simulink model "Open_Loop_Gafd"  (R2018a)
settings: Solver=ode45  StartTime=0.0  StopTime=80  RelTol=1e-3  EnableMultiTasking=on
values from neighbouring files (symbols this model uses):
  Cyb = -0.0245    [init.m]    (also in lqr_des.m)
  Cydel = [-0.24668,0.24668, 0.47413,-0.47413,0]/100    [init.m]    (also in lqr_des.m = [-0.24668,0.24668, 0.47413,-0.47413]/100)
  Cza = -0.073    [init.m]
  Czdel = [0.51664,0.51664,0.60478,0.60478,0.06]/100    [init.m]
  d2r = pi/180    (= 0.0174532925199)    [init.m]
  Mass = 198.32    [init.m]    (also in lqr_des.m)
  Qbar = 150    [init.m]    (also in lqr_des.m)
  r2d = 180/pi    (= 57.2957795131)    [init.m]    (also in pl.m)
  Sref = 79.069    [init.m]    (also in lqr_des.m)
  V0 = 822.8    [init.m]
undefined symbols (not defined in the file or in its folder): Abfp, Afla, Ardr, Avf, Bbfp, Bfla, Brdr, Bvf, Cbfp, Cfla, Crdr, Cvf, Dbfp, Dfla, Drdr, Dvf, K4axmix, Kpr, Kq

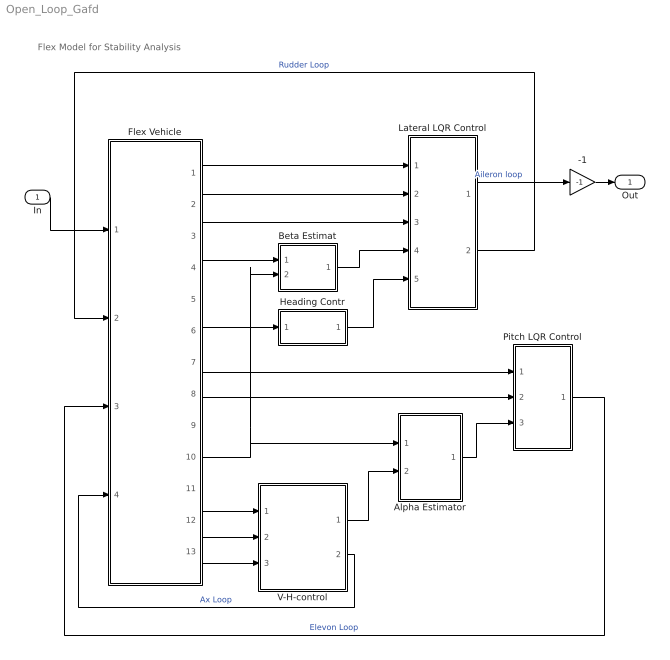
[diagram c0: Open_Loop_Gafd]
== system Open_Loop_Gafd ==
  note: Flex Model for Stability Analysis
  In : Inport
  -1 : Gain  Gain=-1
  Alpha Estimator : Subsystem
  Beta Estimat : Subsystem
  Flex Vehicle : Subsystem
  Heading Contr : Subsystem
  Lateral LQR Control : Subsystem
  Pitch LQR Control : Subsystem
  V-H-control : Subsystem
  Out : Outport
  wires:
  Flex Vehicle/2(p) -> Lateral LQR Control/2(p)
  Flex Vehicle/3(r) -> Lateral LQR Control/3(r)
  Flex Vehicle/1(phi) -> Lateral LQR Control/1(phi)
  Flex Vehicle/8(q) -> Pitch LQR Control/2(q)
  Flex Vehicle/7(thet) -> Pitch LQR Control/1(thet)
  Flex Vehicle/4(Ny) -> Beta Estimat/1(Ydd)
  Flex Vehicle/6("chi ") -> Heading Contr/1(chi)
  Flex Vehicle/12(Nz) -> V-H-control/2(Az)
  Flex Vehicle/13(dH) -> V-H-control/3(dH)
  Flex Vehicle/11(V-dot) -> V-H-control/1(Vdot)
  Flex Vehicle/10(delt) -> Beta Estimat/2(delta), Alpha Estimator/1(delta)
  Alpha Estimator/1(alphat) -> Pitch LQR Control/3(alfa)
  V-H-control/1(Zdd-com) -> Alpha Estimator/2(Zdd)
  Beta Estimat/1(bethat) -> Lateral LQR Control/4(bet)
  -1/1 -> Out/1
  V-H-control/2(Throtle) -> Flex Vehicle/4(Ax-cmd)  "Ax Loop"
  Pitch LQR Control/1(dQ) -> Flex Vehicle/3(dQ)  "Elevon Loop"
  Lateral LQR Control/2(dR) -> Flex Vehicle/2(dR)  "Rudder Loop"
  Heading Contr/1(phi-cmd) -> Lateral LQR Control/5(ph-cmd)
  In/1 -> Flex Vehicle/1(dP)
  Lateral LQR Control/1(dP) -> -1/1  "Aileron loop"

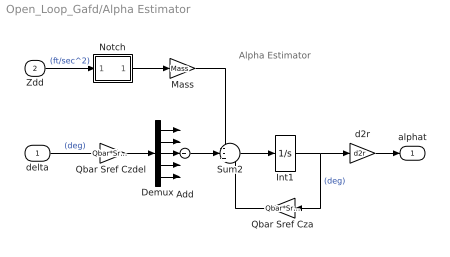
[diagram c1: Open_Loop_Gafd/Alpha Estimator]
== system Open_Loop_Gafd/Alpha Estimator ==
  note: Alpha Estimator
  delta : Inport
  Zdd : Inport  Port=2
  Add : Sum  Inputs=+++++
  Demux : Demux  Outputs=5
  Int1 : Integrator
  Mass : Gain  Gain=Mass
  Notch : Subsystem
  Qbar Sref Cza : Gain  Gain=Qbar*Sref*Cza
  "Qbar Sref Czdel " : Gain  Gain=Qbar*Sref*Czdel
  Sum2 : Sum  Inputs=--+
  d2r : Gain  Gain=d2r
  alphat : Outport
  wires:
  Demux/5 -> Add/5
  Demux/4 -> Add/4
  Demux/3 -> Add/3
  Demux/2 -> Add/2
  Demux/1 -> Add/1
  "Qbar Sref Czdel "/1 -> Demux/1
  delta/1 -> "Qbar Sref Czdel "/1  "(deg)"
  Sum2/1 -> Int1/1
  Int1/1 -> d2r/1, Qbar Sref Cza/1  "(deg)"
  Qbar Sref Cza/1 -> Sum2/3
  Mass/1 -> Sum2/1
  d2r/1 -> alphat/1
  Add/1 -> Sum2/2
  Zdd/1 -> Notch/1(in)  "(ft/sec^2)"
  Notch/1(ou) -> Mass/1

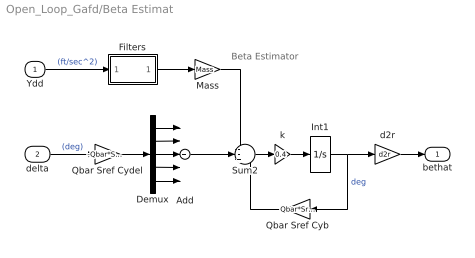
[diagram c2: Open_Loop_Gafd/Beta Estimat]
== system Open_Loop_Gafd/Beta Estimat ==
  note: Beta Estimator
  Ydd : Inport
  delta : Inport  Port=2
  Add : Sum  Inputs=+++++
  Demux : Demux  Outputs=5
  Filters : Subsystem
  Int1 : Integrator
  Mass : Gain  Gain=Mass
  Qbar Sref Cyb : Gain  Gain=Qbar*Sref*Cyb
  Qbar Sref Cydel : Gain  Gain=-Qbar*Sref*Cydel
  Sum2 : Sum  Inputs=--+
  d2r : Gain  Gain=d2r
  k : Gain  Gain=0.4
  bethat : Outport
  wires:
  Filters/1(Ou) -> Mass/1
  Demux/5 -> Add/5
  Demux/4 -> Add/4
  Demux/3 -> Add/3
  Demux/2 -> Add/2
  Demux/1 -> Add/1
  Qbar Sref Cydel/1 -> Demux/1
  delta/1 -> Qbar Sref Cydel/1  "(deg)"
  Sum2/1 -> k/1
  Qbar Sref Cyb/1 -> Sum2/3
  Ydd/1 -> Filters/1(In)  "(ft/sec^2)"
  Mass/1 -> Sum2/1
  d2r/1 -> bethat/1
  Add/1 -> Sum2/2
  Int1/1 -> Qbar Sref Cyb/1, d2r/1  "deg"
  k/1 -> Int1/1

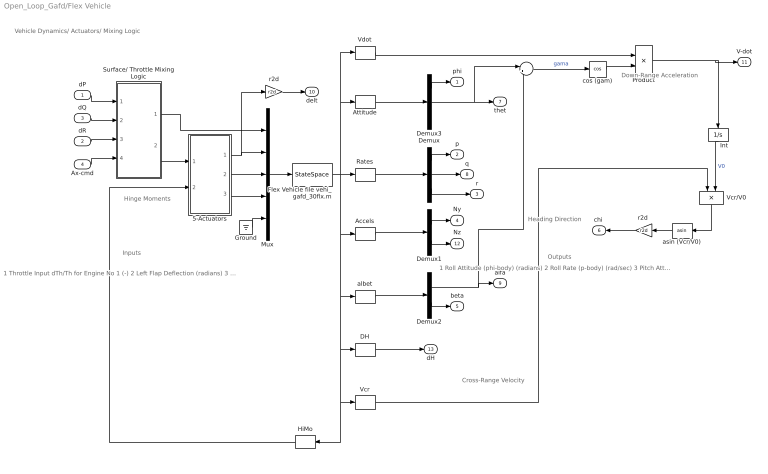
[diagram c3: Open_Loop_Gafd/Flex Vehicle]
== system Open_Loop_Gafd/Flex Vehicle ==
  note: Vehicle Dynamics/ Actuators/ Mixing Logic
  note: Cross-Range Velocity
  note: Heading Direction
  note: Down-Range Acceleration
  note: Outputs
  note: Inputs
  note: 1 Throttle Input dTh/Th for Engine No 1 (-) 2 Left Flap Deflection (radians) 3 Right Flap Deflection (radians) 4 Left Rudder Deflection (radians) 5 Right Rudder Deflection (radians) 6 Body Flap Deflection (radians) 7 Left Flap Velocity (rad/sec) 8 Right Flap Velocity (rad/sec) 9 Left Rudder Velocity (rad/sec) 10 Right Rudder Velocity (rad/sec) 11 Body Flap Velocity (rad/sec) 12 Left Flap Acceleration (rad/s^2) 13 Right Flap Acceleration (rad/s^2) 14 Left Rudder Acceleration (rad/s^2) 15 Right Rudder Acceleration (rad/s^2) 16 Body Flap Acceleration (rad/s^2) 17 Wind Gust Azim, Elev Angles=(45.0 90.0) (deg)
  note: 1 Roll Attitude (phi-body) (radians) 2 Roll Rate (p-body) (rad/sec) 3 Pitch Attitude (thet-bdy) (radians) 4 Pitch Rate (q-body) (rad/sec) 5 Yaw Attitude (psi-body) (radians) 6 Yaw Rate (r-body) (rad/sec) 7 Angle of attack, alfa, (radians) 8 Angle of sideslip, beta, (radian) 9 Change in Altitude, delta-h, (feet) 10 Forward Acceleration (V-dot) (ft/sec) 11 Cross Range Velocity (Vcr) (ft/sec) 12 Rate-Gyro # 1, Roll Rate (Body) (rad/sec) 13 Rate-Gyro # 2, Pitch Rate (Body) (rad/sec) 14 Rate-Gyro # 3, Yaw Rate (Body) (rad/sec) 15 Accelerom # 1, (along Y), (ft/sec^2) Translat. Acceler 16 Accelerom # 2, (along Z), (ft/sec^2) Translat. Acceler 17 Hinge Moment for Aero Surface # 1, (ft-lb) 18 Hinge Moment for Aero Surface # 2, (ft-lb) 19 Hinge Moment for Aero Surface # 3, (ft-lb) 20 Hinge Moment for Aero Surface # 4, (ft-lb) 21 Hinge Moment for Aero Surface # 5, (ft-lb)
  note: Hinge Moments
  dP : Inport
  dR : Inport  Port=2
  dQ : Inport  Port=3
  Ax-cmd : Inport  Port=4
  "    " : Sum  Inputs=|+-
  5-Actuators : Subsystem
  Accels : Selector  InputPortWidth=21  IndexOptions=Index vector (dialog)  Indices=[15,16]  OutputSizes=1
  Attitude : Selector  InputPortWidth=21  IndexOptions=Index vector (dialog)  Indices=[1,3,5]  OutputSizes=1
  DH : Selector  InputPortWidth=21  IndexOptions=Index vector (dialog)  Indices=[9]  OutputSizes=1
  Demux : Demux  Outputs=3
  Demux1 : Demux  Outputs=2
  Demux2 : Demux  Outputs=2
  Demux3 : Demux  Outputs=3
  Flex Vehicle file vehi_gafd_30flx.m : StateSpace  A=Avf  B=Bvf  C=Cvf  D=Dvf  InitialCondition=0
  Ground : Ground
  HiMo : Selector  InputPortWidth=21  IndexOptions=Index vector (dialog)  Indices=[17:21]  OutputSizes=1
  Int : Integrator  InitialCondition=V0
  Mux : Mux  Inputs=[1, 5,5,5, 1]
  Product : Product
  Rates : Selector  InputPortWidth=21  IndexOptions=Index vector (dialog)  Indices=[12:14]  OutputSizes=1
  Surface/ Throttle Mixing Logic : Subsystem
  Vcr : Selector  InputPortWidth=21  IndexOptions=Index vector (dialog)  Indices=[11]  OutputSizes=1
  Vcr/V0 : Product  Inputs=*/
  Vdot : Selector  InputPortWidth=21  IndexOptions=Index vector (dialog)  Indices=[10]  OutputSizes=1
  albet : Selector  InputPortWidth=21  IndexOptions=Index vector (dialog)  Indices=[7,8]  OutputSizes=1
  asin (Vcr/V0) : Trigonometry  Operator=asin
  cos (gam) : Trigonometry  Operator=cos
  r2d : Gain  Gain=r2d
  "r2d " : Gain  Gain=r2d
  phi : Outport
  p : Outport  Port=2
  r : Outport  Port=3
  Ny : Outport  Port=4
  beta : Outport  Port=5
  "chi " : Outport  Port=6
  thet : Outport  Port=7
  q : Outport  Port=8
  alfa : Outport  Port=9
  delt : Outport  Port=10
  V-dot : Outport  Port=11
  Nz : Outport  Port=12
  dH : Outport  Port=13
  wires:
  Vcr/1 -> Vcr/V0/1
  Vdot/1 -> Product/1
  cos (gam)/1 -> Product/2
  DH/1 -> dH/1
  Demux3/1 -> phi/1
  Demux3/2 -> thet/1, "    "/1
  Attitude/1 -> Demux3/1
  Demux2/2 -> beta/1
  Demux2/1 -> alfa/1, "    "/2
  albet/1 -> Demux2/1
  Demux1/2 -> Nz/1
  Demux1/1 -> Ny/1
  Accels/1 -> Demux1/1
  Demux/3 -> r/1
  Demux/2 -> q/1
  Demux/1 -> p/1
  HiMo/1 -> 5-Actuators/2(HM)
  Flex Vehicle file vehi_gafd_30flx.m/1 -> Rates/1, Attitude/1, Vdot/1, Accels/1, albet/1, DH/1, HiMo/1, Vcr/1
  Rates/1 -> Demux/1
  5-Actuators/2(del-dot) -> Mux/3
  5-Actuators/3(del-ddot) -> Mux/4
  5-Actuators/1(delta) -> r2d/1, Mux/2
  Surface/ Throttle Mixing Logic/2(delta) -> 5-Actuators/1(del-cmd)
  "    "/1 -> cos (gam)/1  "gama"
  Int/1 -> Vcr/V0/2  "V0"
  Product/1 -> Int/1, V-dot/1
  asin (Vcr/V0)/1 -> "r2d "/1
  Vcr/V0/1 -> asin (Vcr/V0)/1
  "r2d "/1 -> "chi "/1
  r2d/1 -> delt/1
  Ax-cmd/1 -> Surface/ Throttle Mixing Logic/4(Ax)
  dR/1 -> Surface/ Throttle Mixing Logic/3(yaw)
  dQ/1 -> Surface/ Throttle Mixing Logic/2(ptch)
  dP/1 -> Surface/ Throttle Mixing Logic/1(roll)
  Surface/ Throttle Mixing Logic/1(Throt) -> Mux/1
  Mux/1 -> Flex Vehicle file vehi_gafd_30flx.m/1
  Ground/1 -> Mux/5

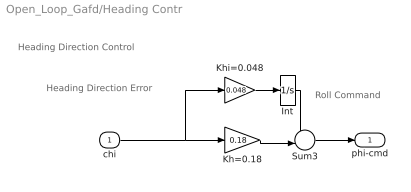
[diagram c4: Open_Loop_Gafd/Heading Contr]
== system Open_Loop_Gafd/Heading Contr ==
  note: Roll Command
  note: Heading Direction Control
  note: Heading Direction Error
  chi : Inport
  Int : Integrator
  Kh=0.18 : Gain  Gain=0.18
  Khi=0.048 : Gain  Gain=0.048
  Sum3 : Sum  Inputs=--|
  phi-cmd : Outport
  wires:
  Khi=0.048/1 -> Int/1
  Kh=0.18/1 -> Sum3/2
  Int/1 -> Sum3/1
  Sum3/1 -> phi-cmd/1
  chi/1 -> Kh=0.18/1, Khi=0.048/1

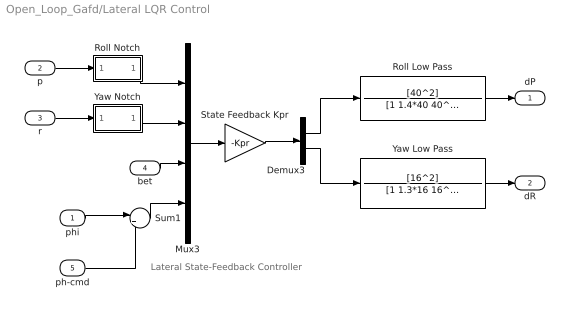
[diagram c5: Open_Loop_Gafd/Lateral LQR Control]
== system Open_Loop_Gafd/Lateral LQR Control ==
  note: Lateral State-Feedback Controller
  phi : Inport
  p : Inport  Port=2
  r : Inport  Port=3
  bet : Inport  Port=4
  ph-cmd : Inport  Port=5
  Demux3 : Demux  Outputs=2
  Mux3 : Mux
  Roll Low Pass : TransferFcn  Numerator=[40^2]  Denominator=[1 1.4*40 40^2]
  Roll Notch : Subsystem
  State Feedback Kpr : Gain  Gain=-Kpr  Multiplication=Matrix(K*u) (u vector)
  Sum1 : Sum  Inputs=|+-
  Yaw Low Pass : TransferFcn  Numerator=[16^2]  Denominator=[1 1.3*16 16^2]
  Yaw Notch : Subsystem
  dP : Outport
  dR : Outport  Port=2
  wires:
  Roll Low Pass/1 -> dP/1
  Demux3/2 -> Yaw Low Pass/1
  r/1 -> Yaw Notch/1(In)
  Roll Notch/1(ou) -> Mux3/1
  ph-cmd/1 -> Sum1/2
  phi/1 -> Sum1/1
  Sum1/1 -> Mux3/4
  Demux3/1 -> Roll Low Pass/1
  bet/1 -> Mux3/3
  p/1 -> Roll Notch/1(in)
  Mux3/1 -> State Feedback Kpr/1
  State Feedback Kpr/1 -> Demux3/1
  Yaw Low Pass/1 -> dR/1
  Yaw Notch/1(Ot) -> Mux3/2

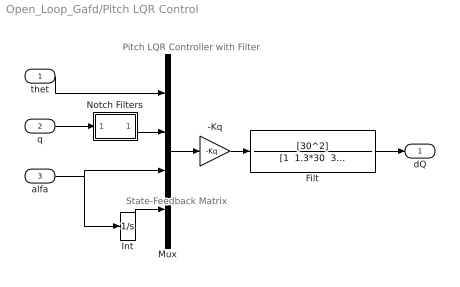
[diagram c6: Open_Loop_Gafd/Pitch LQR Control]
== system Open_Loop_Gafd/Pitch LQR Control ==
  note: State-Feedback Matrix
  note: Pitch LQR Controller with Filter
  thet : Inport
  q : Inport  Port=2
  alfa : Inport  Port=3
  -Kq : Gain  Gain=-Kq  Multiplication=Matrix(K*u)
  Filt : TransferFcn  Numerator=[30^2]  Denominator="[1  1.3*30  30^2]"
  Int : Integrator
  Mux : Mux
  Notch Filters : Subsystem
  dQ : Outport
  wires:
  Filt/1 -> dQ/1
  Notch Filters/1(ou) -> Mux/2
  alfa/1 -> Int/1, Mux/3
  thet/1 -> Mux/1
  q/1 -> Notch Filters/1(in)
  -Kq/1 -> Filt/1
  Int/1 -> Mux/4
  Mux/1 -> -Kq/1

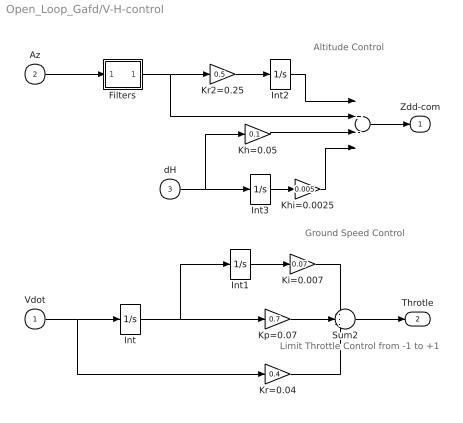
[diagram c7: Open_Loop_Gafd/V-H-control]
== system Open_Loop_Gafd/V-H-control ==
  note: Limit Throttle Control from -1 to +1
  note: Ground Speed Control
  note: Altitude Control
  Vdot : Inport
  Az : Inport  Port=2
  dH : Inport  Port=3
  "  " : Sum  Inputs=++--
  Filters : Subsystem
  Int{,1..3} (4 alike) : Integrator
  Kh=0.05 : Gain  Gain=0.1
  Khi=0.0025 : Gain  Gain=0.005
  Ki=0.007 : Gain  Gain=0.07
  Kp=0.07 : Gain  Gain=0.7
  Kr2=0.25 : Gain  Gain=0.5
  Kr=0.04 : Gain  Gain=0.4
  Sum2 : Sum  Inputs=---
  Zdd-com : Outport
  Throtle : Outport  Port=2
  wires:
  Khi=0.0025/1 -> "  "/4
  Int3/1 -> Khi=0.0025/1
  "  "/1 -> Zdd-com/1
  Int2/1 -> "  "/1
  Kr2=0.25/1 -> Int2/1
  Kh=0.05/1 -> "  "/3
  dH/1 -> Kh=0.05/1, Int3/1
  Int/1 -> Int1/1, Kp=0.07/1
  Int1/1 -> Ki=0.007/1
  Ki=0.007/1 -> Sum2/1
  Kp=0.07/1 -> Sum2/2
  Kr=0.04/1 -> Sum2/3
  Sum2/1 -> Throtle/1
  Vdot/1 -> Kr=0.04/1, Int/1
  Filters/1(ou) -> "  "/2, Kr2=0.25/1
  Az/1 -> Filters/1(in)

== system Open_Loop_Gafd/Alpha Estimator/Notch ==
  note: Notch Filters
  in : Inport
  Notch 79 rad : TransferFcn  Numerator="[1  0.03*79  79^2]"  Denominator="[1  0.4*79  79^2]"
  ou : Outport
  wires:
  in/1 -> Notch 79 rad/1
  Notch 79 rad/1 -> ou/1

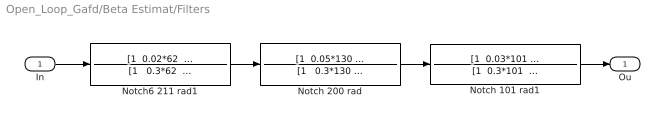
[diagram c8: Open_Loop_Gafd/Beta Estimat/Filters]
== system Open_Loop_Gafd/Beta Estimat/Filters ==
  In : Inport
  Notch 101 rad1 : TransferFcn  Numerator="[1  0.03*101  101^2]"  Denominator="[1  0.3*101  101^2]"
  Notch 200 rad : TransferFcn  Numerator="[1  0.05*130  130^2]"  Denominator="[1   0.3*130  130^2]"
  Notch6 211 rad1 : TransferFcn  Numerator="[1  0.02*62  62.7^2]"  Denominator="[1   0.3*62  62.7^2]"
  Ou : Outport
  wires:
  In/1 -> Notch6 211 rad1/1
  Notch6 211 rad1/1 -> Notch 200 rad/1
  Notch 101 rad1/1 -> Ou/1
  Notch 200 rad/1 -> Notch 101 rad1/1

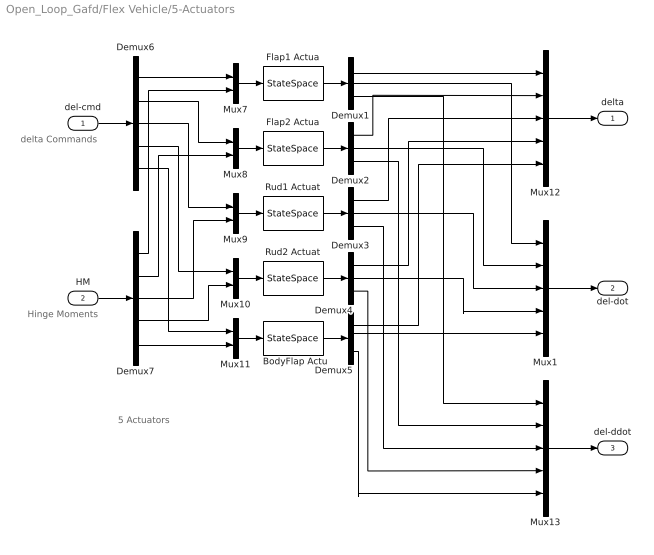
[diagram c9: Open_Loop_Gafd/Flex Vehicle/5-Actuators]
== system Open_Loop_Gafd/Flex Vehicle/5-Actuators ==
  note: delta Commands
  note: Hinge Moments
  note: 5 Actuators
  del-cmd : Inport
  HM : Inport  Port=2
  BodyFlap Actu : StateSpace  A=Abfp  B=Bbfp  C=Cbfp  D=Dbfp  InitialCondition=0
  Demux{1..5} (5 alike) : Demux  Outputs=3
  Demux6 : Demux  Outputs=5
  Demux7 : Demux  Outputs=5
  Flap1 Actua : StateSpace  A=Afla  B=Bfla  C=Cfla  D=Dfla  InitialCondition=0
  Flap2 Actua : StateSpace  A=Afla  B=Bfla  C=Cfla  D=Dfla  InitialCondition=0
  Mux1 : Mux  Inputs=5
  Mux{7..11} (5 alike) : Mux  Inputs=2
  Mux12 : Mux  Inputs=5
  Mux13 : Mux  Inputs=5
  Rud1 Actuat : StateSpace  A=Ardr  B=Brdr  C=Crdr  D=Drdr  InitialCondition=0
  Rud2 Actuat : StateSpace  A=Ardr  B=Brdr  C=Crdr  D=Drdr  InitialCondition=0
  delta : Outport
  del-dot : Outport  Port=2
  del-ddot : Outport  Port=3
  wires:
  Mux1/1 -> del-dot/1
  Demux5/3 -> Mux13/5
  Demux5/2 -> Mux1/5
  Mux13/1 -> del-ddot/1
  HM/1 -> Demux7/1
  Demux4/2 -> Mux1/4
  Demux3/2 -> Mux1/3
  Demux2/2 -> Mux1/2
  del-cmd/1 -> Demux6/1
  Mux12/1 -> delta/1
  Demux1/2 -> Mux1/1
  Demux1/3 -> Mux13/1
  Demux2/3 -> Mux13/2
  Demux3/3 -> Mux13/3
  Demux4/3 -> Mux13/4
  Demux5/1 -> Mux12/5
  Demux4/1 -> Mux12/4
  Demux3/1 -> Mux12/3
  Demux2/1 -> Mux12/2
  Demux1/1 -> Mux12/1
  Demux7/1 -> Mux7/2
  Demux7/2 -> Mux8/2
  Demux7/3 -> Mux9/2
  Demux7/4 -> Mux10/2
  Demux7/5 -> Mux11/2
  Demux6/5 -> Mux11/1
  Demux6/4 -> Mux10/1
  Demux6/3 -> Mux9/1
  Demux6/2 -> Mux8/1
  Demux6/1 -> Mux7/1
  BodyFlap Actu/1 -> Demux5/1
  Mux11/1 -> BodyFlap Actu/1
  Rud2 Actuat/1 -> Demux4/1
  Mux10/1 -> Rud2 Actuat/1
  Rud1 Actuat/1 -> Demux3/1
  Mux9/1 -> Rud1 Actuat/1
  Flap2 Actua/1 -> Demux2/1
  Mux8/1 -> Flap2 Actua/1
  Flap1 Actua/1 -> Demux1/1
  Mux7/1 -> Flap1 Actua/1

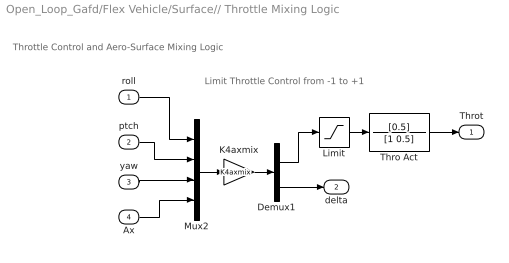
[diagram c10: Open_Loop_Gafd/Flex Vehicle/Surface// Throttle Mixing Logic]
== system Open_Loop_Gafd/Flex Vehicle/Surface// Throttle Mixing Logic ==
  note: Throttle Control and Aero-Surface Mixing Logic
  note: Limit Throttle Control from -1 to +1
  roll : Inport
  ptch : Inport  Port=2
  yaw : Inport  Port=3
  Ax : Inport  Port=4
  Demux1 : Demux  Outputs=[1, 5]
  K4axmix : Gain  Gain=K4axmix  Multiplication=Matrix(K*u) (u vector)
  Limit : Saturate  UpperLimit=1  LowerLimit=-1
  Mux2 : Mux
  Thro Act : TransferFcn  Numerator=[0.5]  Denominator=[1 0.5]
  Throt : Outport
  delta : Outport  Port=2
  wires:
  ptch/1 -> Mux2/2
  yaw/1 -> Mux2/3
  Ax/1 -> Mux2/4
  roll/1 -> Mux2/1
  Demux1/2 -> delta/1
  Demux1/1 -> Limit/1
  Mux2/1 -> K4axmix/1
  K4axmix/1 -> Demux1/1
  Limit/1 -> Thro Act/1
  Thro Act/1 -> Throt/1

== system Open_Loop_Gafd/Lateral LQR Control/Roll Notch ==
  in : Inport
  Notch 63 rad1 : TransferFcn  Numerator="[1  0.02*62  62.7^2]"  Denominator="[1   0.3*62  62.7^2]"
  ou : Outport
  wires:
  in/1 -> Notch 63 rad1/1
  Notch 63 rad1/1 -> ou/1

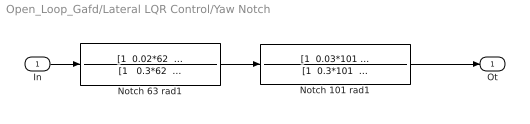
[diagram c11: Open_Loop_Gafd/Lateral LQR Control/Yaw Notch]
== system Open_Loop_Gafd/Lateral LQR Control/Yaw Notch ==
  In : Inport
  Notch 101 rad1 : TransferFcn  Numerator="[1  0.03*101  101^2]"  Denominator="[1  0.3*101  101^2]"
  Notch 63 rad1 : TransferFcn  Numerator="[1  0.02*62  62.7^2]"  Denominator="[1   0.3*62  62.7^2]"
  Ot : Outport
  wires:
  In/1 -> Notch 63 rad1/1
  Notch 63 rad1/1 -> Notch 101 rad1/1
  Notch 101 rad1/1 -> Ot/1

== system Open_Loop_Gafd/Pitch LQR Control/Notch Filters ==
  note: Notch Filters
  in : Inport
  Notch 106 rad : TransferFcn  Numerator="[1  0.02*106  107^2]"  Denominator="[1  0.4*106  107^2]"
  Notch 79 rad : TransferFcn  Numerator="[1  0.02*79  78.5^2]"  Denominator="[1  0.4*79  78.5^2]"
  ou : Outport
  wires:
  in/1 -> Notch 79 rad/1
  Notch 106 rad/1 -> ou/1
  Notch 79 rad/1 -> Notch 106 rad/1

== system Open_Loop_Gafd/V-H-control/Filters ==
  in : Inport
  Notch 106 rad : TransferFcn  Numerator="[1  0.02*106  107^2]"  Denominator="[1  0.4*106  107^2]"
  ou : Outport
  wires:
  in/1 -> Notch 106 rad/1
  Notch 106 rad/1 -> ou/1
